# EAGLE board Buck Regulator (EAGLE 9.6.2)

Size 60 x 40 mm. Coordinates in mm from the lower left corner, seen from the top.
Outline: 0,0 60,0 60,40 0,40 0,0
Copper layers (1*16): Top 0.035mm / dielectric 1.5mm / Bottom 0.035mm
Design rules "default": minimum track width 6mil, minimum drill 0.35mm, track to track 6mil, track to pad 6mil, pad to pad 6mil, via to via 6mil, smd to smd 6mil, copper to edge 40mil, drill to drill 6mil, minimum pad ring 10mil, minimum via ring 8mil, stop-mask expansion 4mil, vias tented up to drill 0mil, thermal gap 10mil

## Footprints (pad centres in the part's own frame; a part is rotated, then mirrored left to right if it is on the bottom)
C1812 = smd 1.9 x 3.4: 1 -1.95,0; 2 1.95,0
C0603 = smd 1.1 x 1: 1 -0.85,0; 2 0.85,0
3,2 = hole 3.2: 0,0
SO-08-EP = smd 0.6 x 1.9: 1 -1.905,-2.9; 2 -0.635,-2.9; 3 0.635,-2.9; 4 1.905,-2.9; 5 1.905,2.9; 6 0.635,2.9; 7 -0.635,2.9; 8 -1.905,2.9 | smd 3.4 x 2.95: 9 0,0
SDR1307-391KL = smd 14 x 4.75: 1 0,4.6; 2 0,-4.6
R0603 = smd 1 x 1.1: 1 -0.85,0; 2 0.85,0
W237-102 = drill 1.194 long: 1 -2.5,-1.27; 2 2.5,-1.27

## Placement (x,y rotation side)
C1  4.7uF/150V  [C1812]  27.94,33.02 0 top
C2  1uF  [C0603]  34.29,16.51 0 top
C3  10nF  [C0603]  19.05,16.51 0 top
C4  4.7nF  [C0603]  15.24,24.13 0 top
C5  4.7uF  [C0603]  21.59,24.13 0 top
C6  4.7uF  [C0603]  29.21,24.13 0 top
H1  MOUNT-HOLE3.2  [3,2]  5,5 0 top
H2  MOUNT-HOLE3.2  [3,2]  5,35 90 top
H3  MOUNT-HOLE3.2  [3,2]  55,35 180 top
IC1  LM5017  [SO-08-EP]  13.97,34.29 270 top
L1  SDR1307-391KL  [SDR1307-391KL]  43.18,30.48 0 top
R1  499k  [R0603]  11.43,16.51 0 top
R2  [R0603]  26.67,16.51 0 top
R3  [R0603]  8.89,24.13 0 top
X1  [W237-102]  50.8,10.16 90 top
X2  [W237-102]  20.32,6.35 0 top

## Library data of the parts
C1-C6 = rcl; SPICEPREFIX: C
H1-H3 = _nanolabs_layout
IC1 = _nanolabs_ic
L1 = _nanolabs_rcl
R1-R3 = rcl; SPICEPREFIX: R
X1 X2 = con-wago-500; MPN: 237-102; OC_FARNELL: unknown; OC_NEWARK: 70K9898

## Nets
+12V: C4.1 C5.1 C6.1 L1.2 R2.2 X2.2
GND: C1.2 C2.2 C5.2 C6.2 IC1.1 IC1.9 R3.1 X1.2 X2.1
N$23: C2.1 IC1.6
N$28: C3.1 IC1.7
N$29: C3.2 IC1.8 L1.1
N$30: C4.2 IC1.5 R2.1 R3.2
N$31: IC1.4 R1.2
VIN_HV: C1.1 IC1.2 IC1.3 R1.1 X1.1

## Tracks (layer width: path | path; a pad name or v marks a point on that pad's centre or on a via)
+12V  (5 unrouted)
GND  (8 unrouted)
N$23  (1 unrouted)
N$28  (1 unrouted)
N$29  (2 unrouted)
N$30  (3 unrouted)
N$31  (1 unrouted)
VIN_HV  (4 unrouted)

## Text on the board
Top: Buck Regulator V0.1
